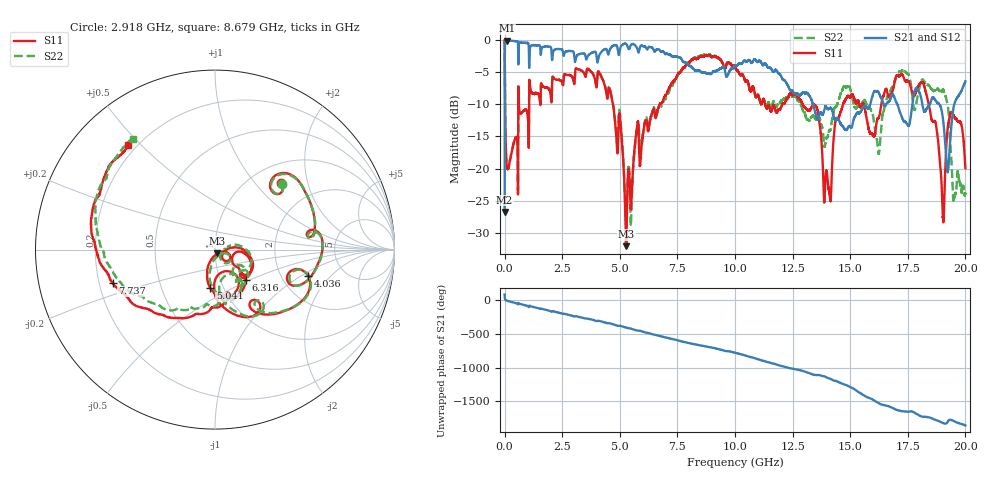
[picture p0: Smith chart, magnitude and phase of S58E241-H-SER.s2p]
!{S58E241}
!Johanson Technology Inc.
!www.johansontechnology.com
!Test Board Conditions:
!Substrate Type  RO4350B
!Substrate Thickness  60 mil
!Substrate Dk  3.66
!TL Type: GCPW
!TL Trace Width  115 mil
!TL Gap  52 mil
!Electrode orientation  Horizontal
!DUT TOPOLOGY	SERIES
!Mounting Pad LxW  55x428 mil
! Created Wed Apr 14 11:34:03 2021
# mhz S ma R 50
! 2 Port Network Data from SP1.SP block
! freq  magS11  angS11  magS21  angS21  magS12  angS12  magS22  angS22
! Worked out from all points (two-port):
!   20001 points, 300 kHz to 20 GHz, reference 50 ohm
!   highest |S21| = -0.05 dB at 106.3 MHz (marker M1); lowest = -26.8 dB at 300 kHz (marker M2)
!   |S21| within 3 dB of the highest: 1.075 GHz to 2.057 GHz (981.7 MHz wide, 62.7 % of centre); 4.057 GHz to 7.697 GHz (3.641 GHz wide, 61.9 % of centre)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
!   lowest |S11| = -32.1 dB at 5.277 GHz (marker M3), VSWR 1.05, Z = 51.3 - j2.15 ohm
!   |S11| at or under -10 dB: 4.703 GHz to 6.726 GHz (2.024 GHz wide, 35.4 % of centre); 12.94 GHz to 14.69 GHz (1.747 GHz wide, 12.7 % of centre); 18.41 GHz to end of sweep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
!   |S22| runs from -28.8 to 0.0 dB; largest |S21 - S12| = 0.013
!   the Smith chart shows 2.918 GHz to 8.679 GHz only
!   S11 on the Smith chart (normalised r, x): 2.918 GHz: 1.36, +1.38; 4.036 GHz: 2.80, -1.18; 5.041 GHz: 0.87, -0.39; 6.316 GHz: 1.32, -0.47; 7.737 GHz: 0.26, -0.15; 8.679 GHz: 0.17, +0.46
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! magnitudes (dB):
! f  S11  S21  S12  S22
! 300 kHz  0.0  -26.8  -26.8  0.0
! 106.3 MHz  -19.9  -0.1  -0.1  -19.9
! 2.918 GHz  -5.7  -1.7  -1.7  -5.7
! 3.334 GHz  -4.7  -2.1  -2.1  -4.7
! 4.036 GHz  -5.3  -3.4  -3.4  -5.2
! 5.041 GHz  -13.3  -1.0  -1.0  -12.9
! 5.277 GHz  -32.1  -0.6  -0.6  -28.0
! 6.316 GHz  -12.4  -1.1  -1.1  -12.5
! 6.667 GHz  -10.6  -1.4  -1.4  -10.9
! 7.737 GHz  -4.4  -3.3  -3.3  -4.3
! 8.679 GHz  -2.4  -5.0  -5.1  -2.3
! 10 GHz  -4.2  -4.0  -4.0  -4.3
! 13.33 GHz  -10.4  -9.5  -9.5  -12.0
! 14.1 GHz  -23.8  -10.6  -10.6  -14.1
! 14.81 GHz  -9.2  -13.9  -14.0  -7.3
! 16.22 GHz  -12.2  -8.1  -8.1  -17.4
! 16.67 GHz  -8.8  -9.6  -9.7  -8.5
! 18.17 GHz  -6.6  -10.6  -10.7  -6.2
! 19.02 GHz  -27.4  -12.1  -12.2  -7.7
! 19.23 GHz  -13.7  -20.6  -20.7  -10.2
! 19.51 GHz  -11.9  -10.1  -10.1  -24.7
! 20 GHz  -20.0  -6.4  -6.4  -23.9
